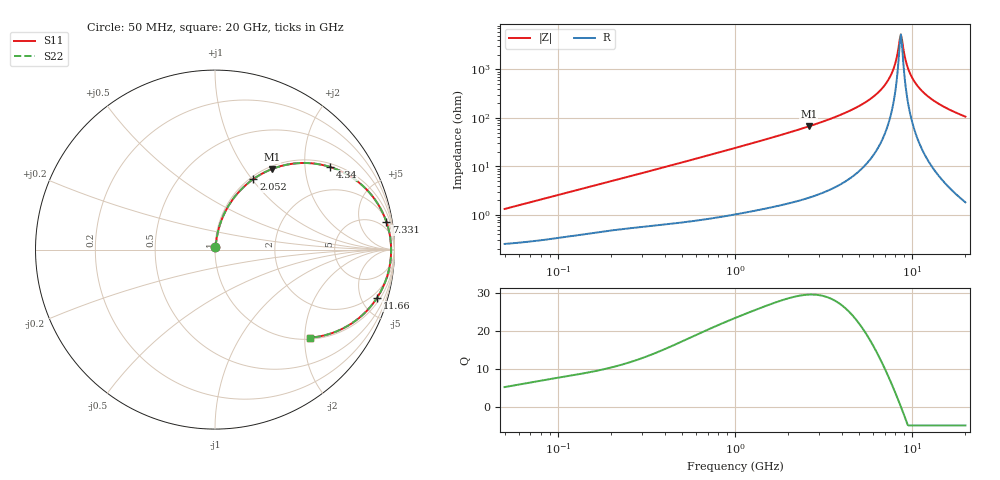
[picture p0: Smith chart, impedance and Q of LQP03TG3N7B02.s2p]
!Murata Part Number: LQP03TG3N7B02
!These Parameters are Measured in Series Mode Connection
!  o--[Z]--o
!Port1  Port2
!  o-------o
!Freq. Start=50[MHz] Stop=20[GHz], 401[Steps]
# Hz S RI R 50
!Freq.(Hz) S11(Real) S11(Imag) S21(Real) S21(Imag) S12(Real) S12(Imag) S22(Real) S22(Imag)
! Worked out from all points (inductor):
!   401 points, 50 MHz to 20 GHz, reference 50 ohm
!   read as one part in series: L = 4.14 nH near 51.52 MHz
!   highest Q = 29.7 at 2.608 GHz (marker M1), where L = 4.09 nH
!   self-resonance near 8.516 GHz
!   S11 on the Smith chart (normalised r, x): 50 MHz: 1.01, +0.03; 2.052 GHz: 1.04, +1.02; 4.34 GHz: 1.11, +2.70; 7.331 GHz: 2, +12; 11.66 GHz: 1.38, -6.57; 20 GHz: 1.04, -2.13
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5e7  0.00269 0.013  0.9973 -0.013  0.9973 -0.013  0.00269 0.013
1.364002e8  0.00511 0.0341  0.9949 -0.0341  0.9949 -0.0341  0.00511 0.0341
3.721004e8  0.0141 0.0883  0.9859 -0.0883  0.9859 -0.0883  0.0141 0.0883
1e9  0.0631 0.2227  0.9369 -0.2227  0.9369 -0.2227  0.0631 0.2227
2.05233e9  0.2142 0.3933  0.7858 -0.3933  0.7858 -0.3933  0.2142 0.3933
2.608132e9  0.3158 0.4483  0.6842 -0.4483  0.6842 -0.4483  0.3158 0.4483
2.728004e9  0.3388 0.4567  0.6612 -0.4567  0.6612 -0.4567  0.3388 0.4567
4.34015e9  0.6407 0.4605  0.3593 -0.4605  0.3593 -0.4605  0.6407 0.4605
5.944466e9  0.8586 0.3197  0.1414 -0.3197  0.1414 -0.3197  0.8586 0.3197
6.701223e9  0.9214 0.2307  0.0786 -0.2307  0.0786 -0.2307  0.9214 0.2307
7.331367e9  0.9553 0.1538  0.0447 -0.1538  0.0447 -0.1538  0.9553 0.1538
7.442007e9  0.9597 0.1403  0.0403 -0.1403  0.0403 -0.1403  0.9597 0.1403
7.901521e9  0.9733 0.085  0.0267 -0.085  0.0267 -0.085  0.9733 0.085
8.389408e9  0.9803 0.0282  0.0197 -0.0282  0.0197 -0.0282  0.9803 0.0282
8.644534e9  0.9814 -0.00053  0.0186 0.00053  0.0186 0.00053  0.9814 -0.00053
8.774992e9  0.9812 -0.0149  0.0188 0.0149  0.0188 0.0149  0.9812 -0.0149
9.316812e9  0.9765 -0.0721  0.0235 0.0721  0.0235 0.0721  0.9765 -0.0721
9.745021e9  0.9686 -0.1143  0.0314 0.1143  0.0314 0.1143  0.9686 -0.1143
1.050288e10  0.9474 -0.1822  0.0526 0.1822  0.0526 0.1822  0.9474 -0.1822
1.166392e10  0.9026 -0.2693  0.0974 0.2693  0.0974 0.2693  0.9026 -0.2693
1.460232e10  0.7626 -0.4105  0.2374 0.4105  0.2374 0.4105  0.7626 -0.4105
2e10  0.5313 -0.4905  0.4687 0.4905  0.4687 0.4905  0.5313 -0.4905
